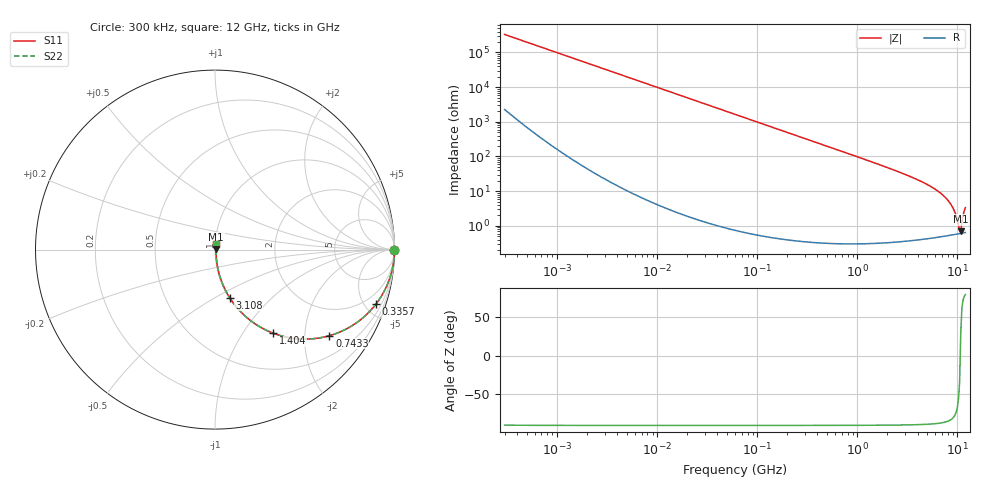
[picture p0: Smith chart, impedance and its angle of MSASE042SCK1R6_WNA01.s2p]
! MSASE042SCK1R6_WNA01  S-PARAMETER MODEL  ( General Type )
! Model Generated by TAIYO YUDEN Corporation (http://www.ty-top.com)
! Version 1.0
! TAIYO YUDEN Control No. 120810
! Copyright(c) 2012 TAIYO YUDEN CO.,LTD. All Rights Reserved.
! Product Description (link to TY-COMPAS)
! https://ds.yuden.co.jp/TYCOMPAS/or/detail?pn=MSASE042SCK1R6AWNA01&u=M
! Products Name : Multilayer Ceramic Capacitors
! Characteristics :
!  Capacitance : 1.6 pF , Rated Voltage : 16V , TCC : CK / C0K
!  Case Size : 0.4 x 0.2 / 0.016 x 0.008 [mm/inch] , Thickness : 0.2 / 0.008 [mm/inch]
!  (Conditions: Temperature = 25 degC , DC Bias Current/Voltage = 0A / 0V)
! External Node Assignments :
!  1  o---| |---o  2
! GND o---------o GND
! Frequency Range : 0.3MHz  -  12000MHz  [ 401 STEP ]
# MHz S RI R 50
! Freq[MHz].  S11 Real  S11 Imag  S21 Real  S21 Imag  S12 Real  S12 Imag  S22 Real  S22 Imag
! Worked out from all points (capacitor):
!   401 points, 300 kHz to 12 GHz, reference 50 ohm
!   read as one part in series: C = 1.61 pF near 316.3 kHz
!   lowest |Z| = 703 mohm at 10.79 GHz (marker M1)
!   series resonance near 10.66 GHz, so ESL is about 140 pH
!   S11 on the Smith chart (normalised r, x): 300 kHz: open; 335.7 MHz: 1.01, -5.90; 743.3 MHz: 1.01, -2.65; 1.404 GHz: 1.01, -1.39; 3.108 GHz: 1.01, -0.58; 12 GHz: 1.01, +0.07
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0.3  1 -0.000303  2.17e-06 0.000303  2.17e-06 0.000303  1 -0.000303
1.769972  1 -0.00179  4.94e-06 0.00179  4.94e-06 0.00179  1 -0.00179
10.44266  0.9999 -0.0105  0.000115 0.0105  0.000115 0.0105  0.9999 -0.0105
60  0.9963 -0.0603  0.00368 0.0603  0.00368 0.0603  0.9963 -0.0603
151.6462  0.977 -0.1495  0.023 0.1495  0.023 0.1495  0.977 -0.1495
335.7268  0.8966 -0.3039  0.1034 0.3039  0.1034 0.3039  0.8966 -0.3039
353.9943  0.8863 -0.3168  0.1137 0.3168  0.1137 0.3168  0.8863 -0.3168
743.2595  0.6375 -0.4796  0.3625 0.4796  0.3625 0.4796  0.6375 -0.4796
1403.667  0.3258 -0.4664  0.6742 0.4664  0.6742 0.4664  0.3258 -0.4664
2088.533  0.1742 -0.3757  0.8258 0.3757  0.8258 0.3757  0.1742 -0.3757
3107.553  0.0814 -0.2674  0.9186 0.2674  0.9186 0.2674  0.0814 -0.2674
5140.631  0.0256 -0.1441  0.9744 0.1441  0.9744 0.1441  0.0256 -0.1441
7254.098  0.0103 -0.0731  0.9897 0.0731  0.9897 0.0731  0.0103 -0.0731
8281.503  0.00756 -0.0478  0.9924 0.0478  0.9924 0.0478  0.00756 -0.0478
8966.534  0.00657 -0.033  0.9934 0.033  0.9934 0.033  0.00657 -0.033
9454.42  0.00616 -0.0232  0.9938 0.0232  0.9938 0.0232  0.00616 -0.0232
10236.47  0.00593 -0.00861  0.9941 0.00861  0.9941 0.00861  0.00593 -0.00861
10511.28  0.00596 -0.00397  0.994 0.00397  0.994 0.00397  0.00596 -0.00397
10793.46  0.00604 0.00352  0.994 -0.00352  0.994 -0.00352  0.00604 0.00352
11083.22  0.00624 0.0115  0.9938 -0.0115  0.9938 -0.0115  0.00624 0.0115
11686.27  0.00697 0.026  0.993 -0.026  0.993 -0.026  0.00697 0.026
12000  0.00744 0.0324  0.9926 -0.0324  0.9926 -0.0324  0.00744 0.0324
